TYPE dut_EXH_Output :
STRUCT
	
	Q300_00				:BOOL;	//	CoolingValve1_Boat
	Q300_01				:BOOL;	//	CoolingValve2_Flange
	Q300_02				:BOOL;
	Q300_03				:BOOL;
	Q300_04				:BOOL;
	Q300_05				:BOOL;
	Q300_06				:BOOL;
	Q300_07				:BOOL;
	Q300_08				:BOOL;	//	APC_auto_close
	Q300_09				:BOOL;	//	APC_pump_on
	Q300_10				:BOOL;
	Q300_11				:BOOL;
	Q300_12				:BOOL;
	Q300_13				:BOOL;
	Q300_14				:BOOL;
	Q300_15				:BOOL;
		
	QEV					:ARRAY[1..1]OF	dut_EX260_SEC ;	//阀岛输出
	
END_STRUCT
END_TYPE
